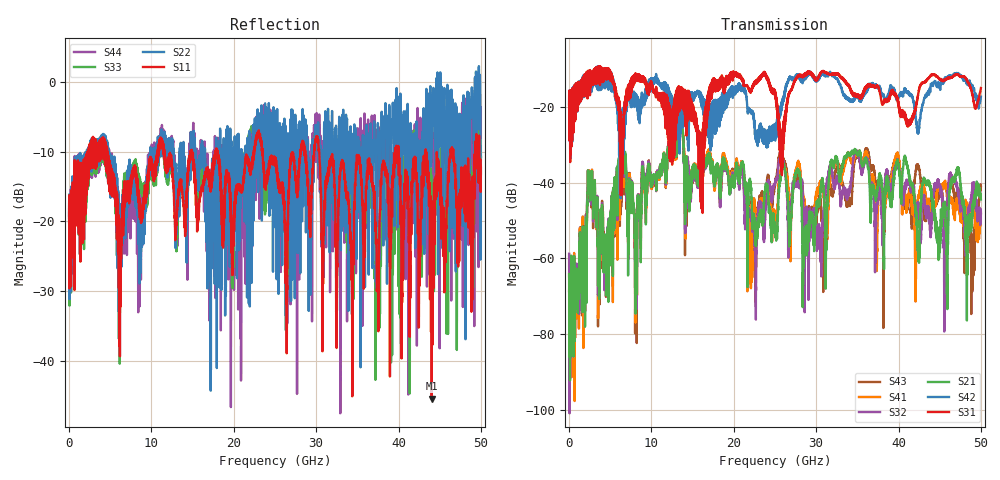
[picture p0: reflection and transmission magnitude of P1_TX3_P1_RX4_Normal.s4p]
!Keysight Technologies,N5225B,MY57041031,A.13.20.10
!Date: Friday, May 31, 2019 11:19:00
!Correction: S11(Full 4 Port(1,2,3,4))
!S12(Full 4 Port(1,2,3,4))
!S13(Full 4 Port(1,2,3,4))
!S14(Full 4 Port(1,2,3,4))
!S21(Full 4 Port(1,2,3,4))
!S22(Full 4 Port(1,2,3,4))
!S23(Full 4 Port(1,2,3,4))
!S24(Full 4 Port(1,2,3,4))
!S31(Full 4 Port(1,2,3,4))
!S32(Full 4 Port(1,2,3,4))
!S33(Full 4 Port(1,2,3,4))
!S34(Full 4 Port(1,2,3,4))
!S41(Full 4 Port(1,2,3,4))
!S42(Full 4 Port(1,2,3,4))
!S43(Full 4 Port(1,2,3,4))
!S44(Full 4 Port(1,2,3,4))
!S4P File: Measurements: <S11,S12,S13,S14>,
!<S21,S22,S23,S24>,
!<S31,S32,S33,S34>,
!<S41,S42,S43,S44>:
# Hz S  dB  R 50.0
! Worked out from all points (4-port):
!   5000 points, 10 MHz to 50 GHz, reference 50 ohm
!   strongest paths, dB at 10 MHz, 12.51 GHz, 25.01 GHz, 37.51 GHz, 50 GHz:
!     S31: -19.3, -27.1, -15.7, -14.5, -15.0
!     S42: -19.4, -19.3, -25.7, -15.1, -17.3
!     S21: -64.1, -26.6, -51.1, -41.2, -44.4
!     S32: -58.8, -26.9, -40.2, -43.0, -48.1
!     S41: -58.9, -26.8, -48.0, -45.9, -48.0
!     S43: -68.6, -27.0, -40.6, -42.5, -40.9
!   lowest |S11| = -45.4 dB at 44.03 GHz (marker M1), VSWR 1.01, Z = 50 + j0.537 ohm
!   |S11| at or under -10 dB: 4.66 GHz to 10.77 GHz (6.106 GHz wide, 79.2 % of centre); 23.49 GHz to 28.08 GHz (4.585 GHz wide, 17.8 % of centre); 30.37 GHz to 39.62 GHz (9.242 GHz wide, 26.4 % of centre)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
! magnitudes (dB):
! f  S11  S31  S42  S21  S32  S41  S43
! 10 MHz  -19.5  -19.3  -19.4  -64.1  -58.8  -58.9  -68.6
! 2.54 GHz  -12.5  -16.9  -15.0  -38.4  -39.0  -38.2  -38.7
! 13.52 GHz  -14.0  -19.7  -26.9  -25.5  -25.7  -25.8  -26.1
! 22.56 GHz  -9.5  -13.7  -26.2  -50.9  -58.0  -45.8  -53.4
! 25.76 GHz  -15.0  -27.3  -20.7  -37.6  -34.2  -37.0  -33.3
! 44.03 GHz  -45.4  -11.4  -14.2  -43.2  -50.1  -46.5  -48.2
! 50 GHz  -12.3  -15.0  -17.3  -44.4  -48.1  -48.0  -40.9
